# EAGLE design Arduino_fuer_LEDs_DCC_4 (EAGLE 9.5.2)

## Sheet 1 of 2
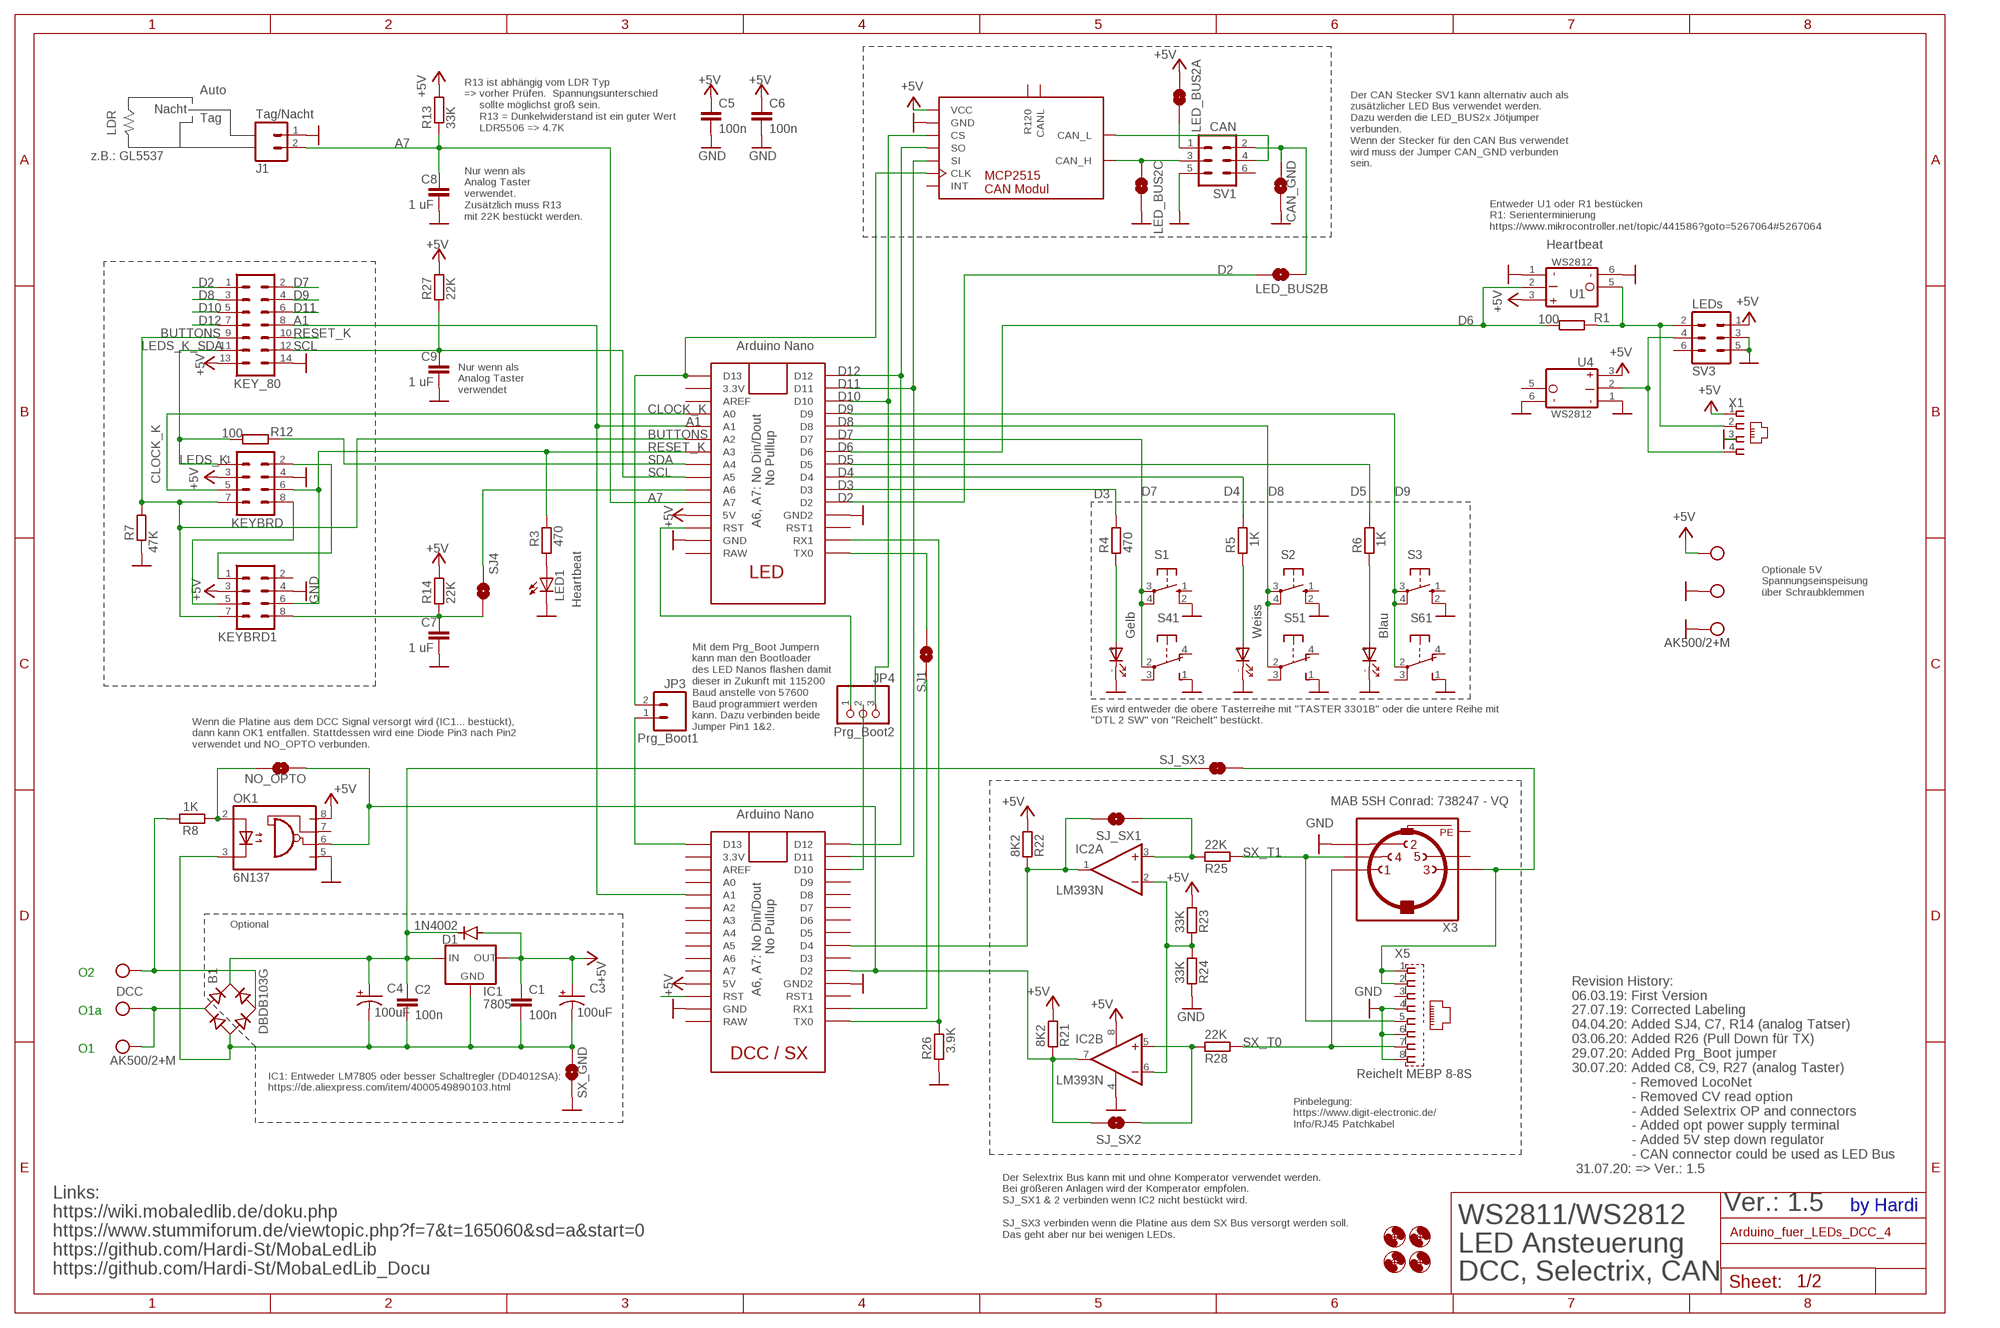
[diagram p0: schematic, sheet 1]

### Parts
B1  DBDB103G  DBDB10G  [DB]
C1  100n  C-EU025-025X050  [C025-025X050]
C2  100n  C-EU025-025X050  [C025-025X050]
C3  100uF  SPARKFUN-CAPACITORS_100UF-25V-20%(PTH)  [SPARKFUN-CAPACITORS_CPOL-RADIAL-100UF-25V]
C4  100uF  SPARKFUN-CAPACITORS_100UF-25V-20%(PTH)  [SPARKFUN-CAPACITORS_CPOL-RADIAL-100UF-25V]
C5  100n  C-EU025-025X050  [C025-025X050]
C6  100n  C-EU025-025X050  [C025-025X050]
C7  1 uF  C-EU025-025X050  [C025-025X050]
C8  1 uF  C-EU025-025X050  [C025-025X050]
C9  1 uF  C-EU025-025X050  [C025-025X050]
CAN2  MCP2515_CAN_MODUL  [MCP2515_CAN_MODUL]
CAN_GND  SOLDERJUMPERNO  [SJ_2S-NO]
D1  1N4002  1N4004  [DO41-10]
H1  MOUNT-HOLE3.0  [3,0]
H2  MOUNT-HOLE3.0  [3,0]
H3  MOUNT-HOLE3.0  [3,0]
H4  MOUNT-HOLE3.0  [3,0]
IC1  7805  78XXS  [78XXS]
IC2  LM393N  [DIL08]
J1  Tag/Nacht  M02PTH  [1X02]
JP3  Prg_Boot1  M02PTH  [1X02]
JP4  Prg_Boot2  PINHD-1X3CB  [1X03-CLEANBIG]
KEY_80  ML14  [ML14]
KEYBRD  CON-HARTING-ML_ML08  [CON-HARTING-ML_ML08]
KEYBRD1  CON-HARTING-ML_ML08  [CON-HARTING-ML_ML08]
LED1  Heartbeat  LED3MM  [LED3MM]
LED_BUS2A  SOLDERJUMPERNO  [SJ_2S-NO]
LED_BUS2B  SOLDERJUMPERNO  [SJ_2S-NO]
LED_BUS2C  SOLDERJUMPERNO  [SJ_2S-NO]
NO_OPTO  SOLDERJUMPERNO  [SJ_2S-NO]
OK1  6N137  [DIL08]
R1  100  R0204/7  [0204/7]
R3  470  R0204/7  [0204/7]
R4  470  R0204/7  [0204/7]
R5  1K  R0204/7  [0204/7]
R6  1K  R0204/7  [0204/7]
R7  47K  R0204/7  [0204/7]
R8  1K  R0204/7  [0204/7]
R12  100  R0204/7  [0204/7]
R13  33K  R0204/7  [0204/7]
R14  22K  R0204/7  [0204/7]
R21  8K2  R-EU_0207/2V  [0207/2V]
R22  8K2  R-EU_0207/2V  [0207/2V]
R23  33K  R-EU_0207/2V  [0207/2V]
R24  33K  R-EU_0207/2V  [0207/2V]
R25  22K  R-EU_0207/2V  [0207/2V]
R26  3.9K  R0204/7  [0204/7]
R27  22K  R0204/7  [0204/7]
R28  22K  R-EU_0207/2V  [0207/2V]
S1  10-XX  [B3F-10XX]
S2  10-XX  [B3F-10XX]
S3  10-XX  [B3F-10XX]
S4  Gelb  SRKL  [SRKL]
S5  Weiss  SRKL  [SRKL]
S6  Blau  SRKL  [SRKL]
SJ1  SOLDERJUMPERNO  [SJ_2S-NO]
SJ4  SOLDERJUMPERNO  [SJ_2S-NO]
SJ_SX1  SOLDERJUMPERNO  [SJ_2S-NO]
SJ_SX2  SOLDERJUMPERNO  [SJ_2S-NO]
SJ_SX3  SOLDERJUMPERNO  [SJ_2S-NO]
SV1  CAN  ML6  [ML6]
SV3  LEDs  ML6  [ML6]
SX_GND  SOLDERJUMPERNO  [SJ_2S-NO]
U1  WS2812_MODUL  [WS2812_LED_MODUL]
U2  LED NANO  NANO  [NANO]
U3  DCC NANO  NANO  [NANO]
U4  WS2812_MODUL  [WS2812_LED_MODUL]
X1  RJ10  [RJ10]
X2  AK500/2+M  [AK500/2+M]
X3  MAB 5SH Conrad: 738247 - VQ  MAB5SH  [MAB5SH]
X4  AK500/2+M  [AK500/2+M]
X5  Reichelt MEBP 8-8S  RJ45_MEBP8-8S  [RJ45_MEBP8-8S]

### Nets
+5V: C1.1 C3.1(+) C5.1 C6.1 CAN2.1(VCC) D1.A IC1.OUT IC2.8(P:V+) KEY_80.13 KEYBRD1.3 KEYBRD.3 LED_BUS2A.1 OK1.8(VCC) R13.2 R14.2 R21.2 R22.2 R23.2 R27.2 SV3.1 U1.3(VDD) U2.5V U3.5V U4.3(VDD) X1.1 X4.2
A1: KEY_80.8 U2.A1 U3.A1
A7: C8.1 J1.2 R13.1 U2.A7
BUTTONS: KEY_80.9 KEYBRD1.7 KEYBRD.7 R7.2 U2.A2
CAN_H: CAN2.9(CAN_H) LED_BUS2C.1 SV1.3
CAN_L: CAN2.8(CAN_L) SV1.4
CLOCK_K: KEYBRD.5 U2.A0
D2: KEY_80.1 LED_BUS2B.1 U2.D2
D3: R4.2 U2.D3
D4: R5.2 U2.D4
D5: R6.2 U2.D5
D6: R1.2 U1.2(DIN) U2.D6
D7: KEY_80.2 S1.3(P) S1.4(P1) S4.2(1:P) U2.D7
D8: KEY_80.3 S2.3(P) S2.4(P1) S5.2(1:P) U2.D8
D9: KEY_80.4 S3.3(P) S3.4(P1) S6.2(1:P) U2.D9
D10: CAN2.3(CS) JP4.3 KEY_80.5 U2.D10
D11: CAN2.5(SI) KEY_80.6 U2.D11 U3.D11
D12: CAN2.4(SO) KEY_80.7 U2.D12 U3.D12
GND: C5.2 C6.2 C7.2 C8.2 C9.2 CAN2.2(GND) CAN_GND.2 IC2.4(P:V-) J1.1 KEY_80.14 KEYBRD1.4 KEYBRD.4 LED1.K(C) LED_BUS2C.2 OK1.5(GND) R7.1 R24.1 R26.1 S1.2(S1) S2.2(S1) S3.2(S1) S4.1(1:S) S4.-(D1:C) S5.1(1:S) S5.-(D1:C) S6.1(1:S) S6.-(D1:C) SV1.5 SV3.3 SV3.5 SX_GND.2 U1.1(GND) U1.6(GND1) U2.GND U2.GND1(GND2) U3.GND U3.GND1(GND2) U4.1(GND) U4.6(GND1) X1.3 X3.2 X4.1 X4.M X5.4 X5.6 X5.8
LEDS_K_SDA: KEY_80.11 KEYBRD.1 R12.2
N$1: SJ1.2 U2.TX0
N$2: R1.1 SV3.2 U1.5(DO) X1.2
N$3: R26.2 U2.RX1 U3.TX0
N$4: R4.1 S4.+(D1:A)
N$5: CAN2.6(CLK) JP3.2 U2.D13
N$6: R5.1 S5.+(D1:A)
N$7: R6.1 S6.+(D1:A)
N$8: IC2.7(B:OUT) NO_OPTO.1 OK1.6(VO) R21.1 SJ_SX2.2 U3.D2
N$9: U3.RST
N$10: LED_BUS2A.2 SV1.1
N$11: SV3.4 U4.2(DIN) X1.4
N$12: B1.AC2 R8.2 X2.2
N$13: B1.AC1 X2.1 X2.M
N$14: B1.+ C2.1 C4.1(+) D1.C IC1.IN SJ_SX3.2
N$15: JP4.1 U2.RST
N$16: IC2.1(A:OUT) R22.1 SJ_SX1.2 U3.D4
N$17: B1.- C1.2 C2.2 C3.2(-) C4.2(-) IC1.GND OK1.3(C) SX_GND.1
N$18: SJ1.1 U3.RX1
N$19: LED1.A R3.1
N$20: JP3.1 U3.D13
N$21: NO_OPTO.2 OK1.2(A) R8.1
N$23: C7.1 KEYBRD1.8 R14.1 SJ4.2
N$24: KEYBRD1.1 KEYBRD.2
N$25: KEYBRD1.5 KEYBRD.8
N$26: SJ_SX3.1 X3.3 X5.1 X5.2
N$27: SJ4.1 U2.A6
N$28: JP4.2 U3.D10
N$29: CAN_GND.1 LED_BUS2B.2 SV1.2
N$38: IC2.2(A:-IN) IC2.6(B:-IN) R23.1 R24.2
N$39: IC2.3(A:+IN) R25.1 SJ_SX1.1
N$42: IC2.5(B:+IN) R28.1 SJ_SX2.1
RESET_K: KEY_80.10 KEYBRD1.6 KEYBRD.6 R3.2 U2.A3
SCL: C9.1 KEY_80.12 R27.1 U2.A5
SDA: R12.1 U2.A4
SX_T0: R28.2 X3.1 X5.7
SX_T1: R25.2 X3.4 X5.5
Unconnected: CAN2.7(INT) CAN2.10(R120) CAN2.11(CANL) KEYBRD1.2 OK1.7(VE) S1.1(S) S2.1(S) S3.1(S) S4.3(1:P) S4.4(1:O) S5.3(1:P) S5.4(1:O) S6.3(1:P) S6.4(1:O) SV1.6 SV3.6 U2.3.3V U2.AREF U2.RAW U2.RST1 U3.3.3V U3.A0 U3.A2 U3.A3 U3.A4 U3.A5 U3.A6 U3.A7 U3.AREF U3.D3 U3.D5 U3.D6 U3.D7 U3.D8 U3.D9 U3.RAW U3.RST1 U4.5(DO) X3.5 X5.3

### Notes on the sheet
- R13 ist abhängig vom LDR Typ
  => vorher Prüfen.  Spannungsunterschied
       sollte möglichst groß sein.
       R13 = Dunkelwiderstand ist ein guter Wert
       LDR5506 => 4.7K
- Der CAN Stecker SV1 kann alternativ auch als
  zusätzlicher LED Bus verwendet werden.
  Dazu werden die LED_BUS2x Jötjumper
  verbunden.
  Wenn der Stecker für den CAN Bus verwendet
  wird muss der Jumper CAN_GND verbunden
  sein.
- Auto
- Nacht
- Tag
- LDR
- z.B.: GL5537
- Nur wenn als
  Analog Taster
  verwendet.
  Zusätzlich muss R13 
  mit 22K bestückt werden.
- Entweder U1 oder R1 bestücken 
  R1: Serienterminierung
  https://www.mikrocontroller.net/topic/441586?goto=5267064#5267064
- Heartbeat
- Nur wenn als
  Analog Taster
  verwendet
- LEDS_K
- A6, A7: No Din/Dout 
              No Pullup
- LED
- Optionale 5V
  Spannungseinspeisung
  über Schraubklemmen
- Es wird entweder die obere Tasterreihe mit "TASTER 3301B" oder die untere Reihe mit 
  "DTL 2 SW" von "Reichelt" bestückt.
- Wenn die Platine aus dem DCC Signal versorgt wird (IC1... bestückt), 
  dann kann OK1 entfallen. Stattdessen wird eine Diode Pin3 nach Pin2
  verwendet und NO_OPTO verbunden.
- Mit dem Prg_Boot Jumpern
  kann man den Bootloader
  des LED Nanos flashen damit
  dieser in Zukunft mit 115200
  Baud anstelle von 57600
  Baud programmiert werden 
  kann. Dazu verbinden beide
  Jumper Pin1 1&2.
- Optional
- O2
- DCC
- A6, A7: No Din/Dout 
              No Pullup
- O1a
- DCC / SX
- O1
- IC1: Entweder LM7805 oder besser Schaltregler (DD4012SA):
  https://de.aliexpress.com/item/4000549890103.html
- Pinbelegung:
  https://www.digit-electronic.de/
  Info/RJ45 Patchkabel
- Der Selextrix Bus kann mit und ohne Komperator verwendet werden.
  Bei größeren Anlagen wird der Komperator empfolen. 
  SJ_SX1 & 2 verbinden wenn IC2 nicht bestückt wird.
  
  SJ_SX3 verbinden wenn die Platine aus dem SX Bus versorgt werden soll.
  Das geht aber nur bei wenigen LEDs.
- Revision History:
  06.03.19: First Version
  27.07.19: Corrected Labeling
  04.04.20: Added SJ4, C7, R14 (analog Tatser)
  03.06.20: Added R26 (Pull Down für TX)
  29.07.20: Added Prg_Boot jumper
  30.07.20: Added C8, C9, R27 (analog Taster)
                 - Removed LocoNet
                 - Removed CV read option
                 - Added Selextrix OP and connectors
                 - Added opt power supply terminal 
                 - Added 5V step down regulator
                 - CAN connector could be used as LED Bus
   31.07.20: => Ver.: 1.5
- Ver.: 1.5 | by Hardi
- Links:
  https://wiki.mobaledlib.de/doku.php
  https://www.stummiforum.de/viewtopic.php?f=7&t=165060&sd=a&start=0
  https://github.com/Hardi-St/MobaLedLib
  https://github.com/Hardi-St/MobaLedLib_Docu
- WS2811/WS2812
  LED Ansteuerung
  DCC, Selectrix, CAN

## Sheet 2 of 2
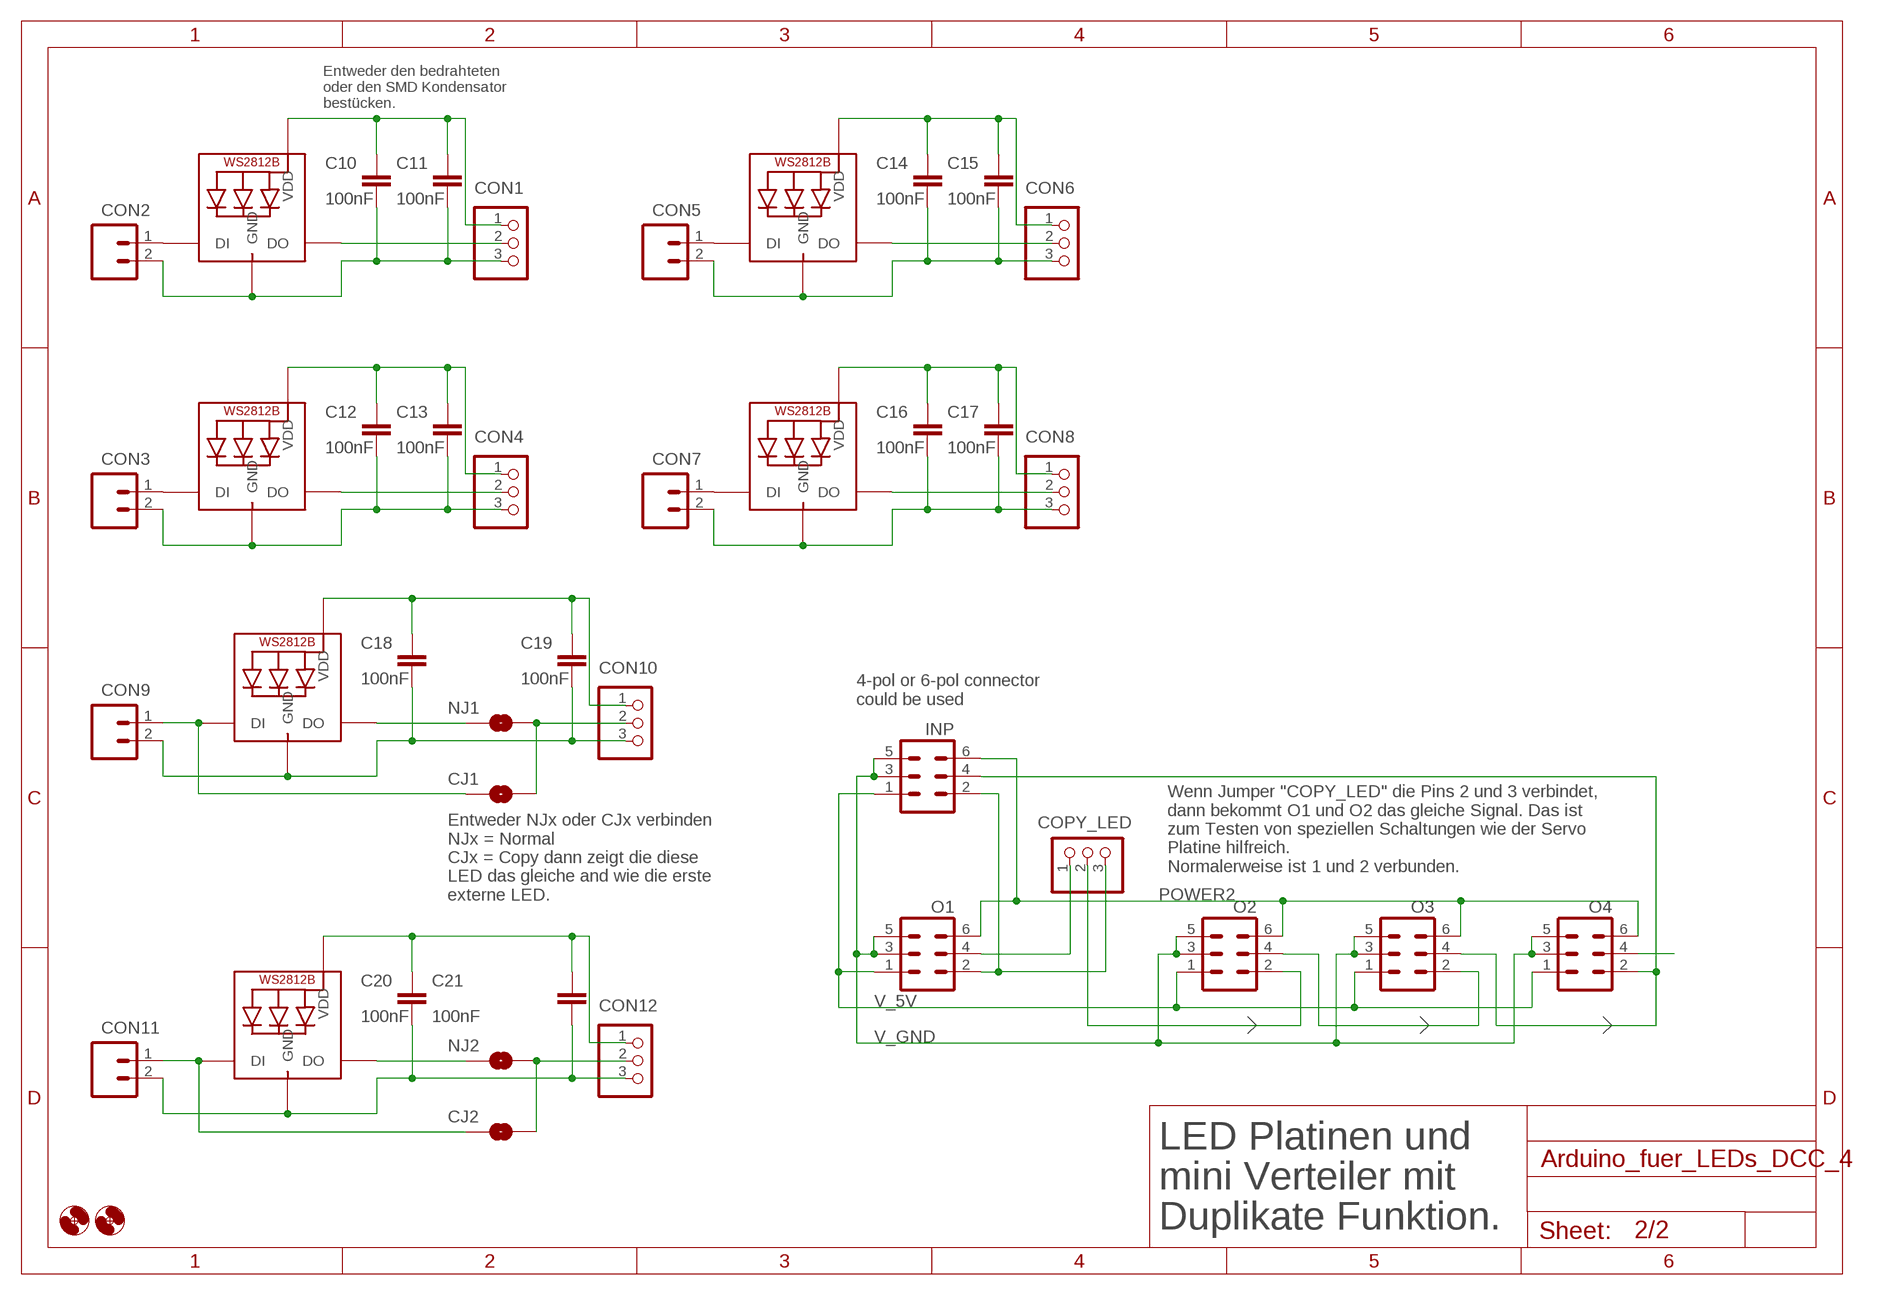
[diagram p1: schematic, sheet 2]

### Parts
C10  100nF  C-EU025-025X050  [C025-025X050]
C11  100nF  C-EUC1206  [C1206]
C12  100nF  C-EU025-025X050  [C025-025X050]
C13  100nF  C-EUC1206  [C1206]
C14  100nF  C-EU025-025X050  [C025-025X050]
C15  100nF  C-EUC1206  [C1206]
C16  100nF  C-EU025-025X050  [C025-025X050]
C17  100nF  C-EUC1206  [C1206]
C18  100nF  C-EU025-025X050  [C025-025X050]
C19  100nF  C-EUC1206  [C1206]
C20  100nF  C-EU025-025X050  [C025-025X050]
C21  100nF  C-EUC1206  [C1206]
CJ1  SOLDERJUMPERNO  [SJ_2S-NO]
CJ2  SOLDERJUMPERNO  [SJ_2S-NO]
CON1  PINHD-1X3CB  [1X03-CLEANBIG]
CON2  M02PTH  [1X02]
CON3  M02PTH  [1X02]
CON4  PINHD-1X3CB  [1X03-CLEANBIG]
CON5  M02PTH  [1X02]
CON6  PINHD-1X3CB  [1X03-CLEANBIG]
CON7  M02PTH  [1X02]
CON8  PINHD-1X3CB  [1X03-CLEANBIG]
CON9  M02PTH  [1X02]
CON10  PINHD-1X3CB  [1X03-CLEANBIG]
CON11  M02PTH  [1X02]
CON12  PINHD-1X3CB  [1X03-CLEANBIG]
COPY_LED  PINHD-1X3CB  [1X03-CLEANBIG]
H5  MOUNT-HOLE3.0  [3,0]
H6  MOUNT-HOLE3.0  [3,0]
INP  ML6  [ML6]
LED2  WS2812B5050  [WS2812B]
LED3  WS2812B5050  [WS2812B]
LED4  WS2812B3535  [LED3535]
LED5  WS2812B3535  [LED3535]
LED6  WS2812B5050  [WS2812B]
LED7  WS2812B3535  [LED3535]
NJ1  SOLDERJUMPERNO  [SJ_2S-NO]
NJ2  SOLDERJUMPERNO  [SJ_2S-NO]
O1  ML6  [ML6]
O2  ML6  [ML6]
O3  ML6  [ML6]
O4  ML6  [ML6]

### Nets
N$22: C10.2 C11.2 CON1.3 CON2.2 LED2.3-GND(GND)
N$30: CON1.2 LED2.2-DOUT(DO)
N$31: C12.2 C13.2 CON3.2 CON4.3 LED3.3-GND(GND)
N$32: C10.1 C11.1 CON1.1 LED2.1-VDD(VDD)
N$33: CON2.1 LED2.4-DIN(DI)
N$34: CON4.2 LED3.2-DOUT(DO)
N$35: C12.1 C13.1 CON4.1 LED3.1-VDD(VDD)
N$36: CON3.1 LED3.4-DIN(DI)
N$37: C14.2 C15.2 CON5.2 CON6.3 LED4.4(GND)
N$40: CON6.2 LED4.3(DO)
N$41: C14.1 C15.1 CON6.1 LED4.2(VDD)
N$43: CON5.1 LED4.1(DI)
N$44: C16.2 C17.2 CON7.2 CON8.3 LED5.4(GND)
N$45: CON8.2 LED5.3(DO)
N$46: C16.1 C17.1 CON8.1 LED5.2(VDD)
N$47: CON7.1 LED5.1(DI)
N$48: C18.2 C19.2 CON9.2 CON10.3 LED6.3-GND(GND)
N$49: LED6.2-DOUT(DO) NJ1.1
N$50: C18.1 C19.1 CON10.1 LED6.1-VDD(VDD)
N$51: CJ1.1 CON9.1 LED6.4-DIN(DI)
N$52: INP.4 O3.4 O4.2
N$53: O4.4
N$54: C20.2 C21.2 CON11.2 CON12.3 LED7.4(GND)
N$55: COPY_LED.2 O2.2
N$56: LED7.3(DO) NJ2.1
N$57: COPY_LED.3 INP.2 O1.2
N$58: O2.4 O3.2
N$59: C20.1 C21.1 CON12.1 LED7.2(VDD)
N$60: COPY_LED.1 O1.4
N$61: CJ2.1 CON11.1 LED7.1(DI)
N$62: CJ2.2 CON12.2 NJ2.2
N$63: CJ1.2 CON10.2 NJ1.2
POWER2: INP.6 O1.6 O2.6 O3.6 O4.6
V_5V: INP.1 O1.1 O2.1 O3.1 O4.1
V_GND: INP.3 INP.5 O1.3 O1.5 O2.3 O2.5 O3.3 O3.5 O4.3 O4.5

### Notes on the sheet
- Entweder den bedrahteten 
  oder den SMD Kondensator 
  bestücken.
- 4-pol or 6-pol connector
  could be used
- Wenn Jumper "COPY_LED" die Pins 2 und 3 verbindet,
  dann bekommt O1 und O2 das gleiche Signal. Das ist
  zum Testen von speziellen Schaltungen wie der Servo 
  Platine hilfreich.
  Normalerweise ist 1 und 2 verbunden.
- Entweder NJx oder CJx verbinden
  NJx = Normal
  CJx = Copy dann zeigt die diese
  LED das gleiche and wie die erste
  externe LED.
- LED Platinen und
  mini Verteiler mit 
  Duplikate Funktion.

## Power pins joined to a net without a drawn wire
PE: X3.PE X3.PE@(PE)

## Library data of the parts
B1 = Arduino_fuer_LEDs_DCC_2:DB?*G: Single Phase 1.0 AMP Glass Passivated Bridge Rectifier Taiwan Semiconductor Co.,Ltd. - TSC Source: http://www.taiwansemi.com/TSCbig5/ezcatfiles/cust/img/img/db101g.pdf http://www.ts.com.tw/db/pictures/modules/PDT/PDT060207001/DBLS201G.pdf
C1 C2 C5-C21 = rcl:C-EU: CAPACITOR, European symbol
C3 C4 = Sound_MP3-TF-16P_and_WS2811:SPARKFUN-CAPACITORS_100UF-25V-20%(PTH): CAP-08439; PROD_ID: CAP-08439
CAN2 = Arduino_fuer_LEDs_DCC_2_All:MCP2515_CAN_MODUL: MCP2515 CAN Modul
CAN_GND CJ1 CJ2 LED_BUS2A LED_BUS2B LED_BUS2C NJ1 NJ2 NO_OPTO SJ1 SJ4 SJ_SX1-SJ_SX3 SX_GND = SparkFun-Retired:SOLDERJUMPER: Solder Jumper
CON1 CON4 CON6 CON8 CON10 CON12 COPY_LED JP4 = adafruit:PINHD-1X3: PIN HEADER
CON2 CON3 CON5 CON7 CON9 CON11 J1 JP3 = SparkFun-Connectors:M02: Standard 2-pin 0.1" header. Use with
D1 = diode:1N4004: DIODE
H1-H6 = holes:MOUNT-HOLE: MOUNTING HOLE with drill center marker
IC1 = v-reg:78XXS: VOLTAGE REGULATOR
IC2 = linear:LM393: COMPARATOR
INP O1-O4 = con-harting-ml:ML6: HARTING; OC_FARNELL: unknown; OC_NEWARK: unknown
KEY_80 = Arduino_fuer_LEDs_DCC_2:ML14: HARTING; OC_FARNELL: unknown; OC_NEWARK: unknown
KEYBRD KEYBRD1 = PushButtonAction_4017_2:CON-HARTING-ML_ML08: Modified by Hardi; OC_FARNELL: unknown; OC_NEWARK: unknown
LED1 = Arduino_fuer_LEDs_DCC_2:LED: LED
LED2-LED7 = adafruit:WS2812B
OK1 = Arduino_fuer_LEDs_DCC_2:6N137: MOTOROLA OPTO COUPLER; MPN: 6N137; OC_FARNELL: 1328376; OC_NEWARK: 52M1895
R1 R3-R8 R12-R14 R26 R27 = Arduino_fuer_LEDs_DCC_2:R: RESISTOR, European symbol; SPICEMODEL: NONE; SPICEPREFIX: R
R21-R25 R28 = rcl:R-EU_: RESISTOR, European symbol
S1-S3 = switch-omron:10-XX: OMRON SWITCH; MPN: B3F-1000; OC_FARNELL: 176432; OC_NEWARK: 36M3542
S4-S6 = switch-misc:SRKL: SWITCH
SV1 SV3 = Arduino_fuer_LEDs_DCC_2:ML6: HARTING; OC_FARNELL: unknown; OC_NEWARK: unknown
U1 U4 = Arduino_fuer_LEDs_DCC_2_All:WS2812_MODUL: WS2812 Modul mit Winkelsteckern (by Hardi)
U2 U3 = Arduino_fuer_LEDs_DCC_2:NANO: Arduino Nano
X1 = RJ10:RJ10: RJ10 Connector "C:\Dat\Märklin\Schaltpläne\Allgemein\RJ10_Stecker_Layout.docx" ...; OC_FARNELL: unknown; OC_NEWARK: unknown
X2 X4 = Arduino_fuer_LEDs_DCC_2:AK500/2+M
X3 = con-hirschmann:MAB5SH: Female CONNECTOR 5 pins 90 deg. with shield, horizontal (DIN 41524); OC_FARNELL: 809883; OC_NEWARK: unknown
X5 = RJ45_Reichelt:RJ45_MEBP8-8S: AMP connector

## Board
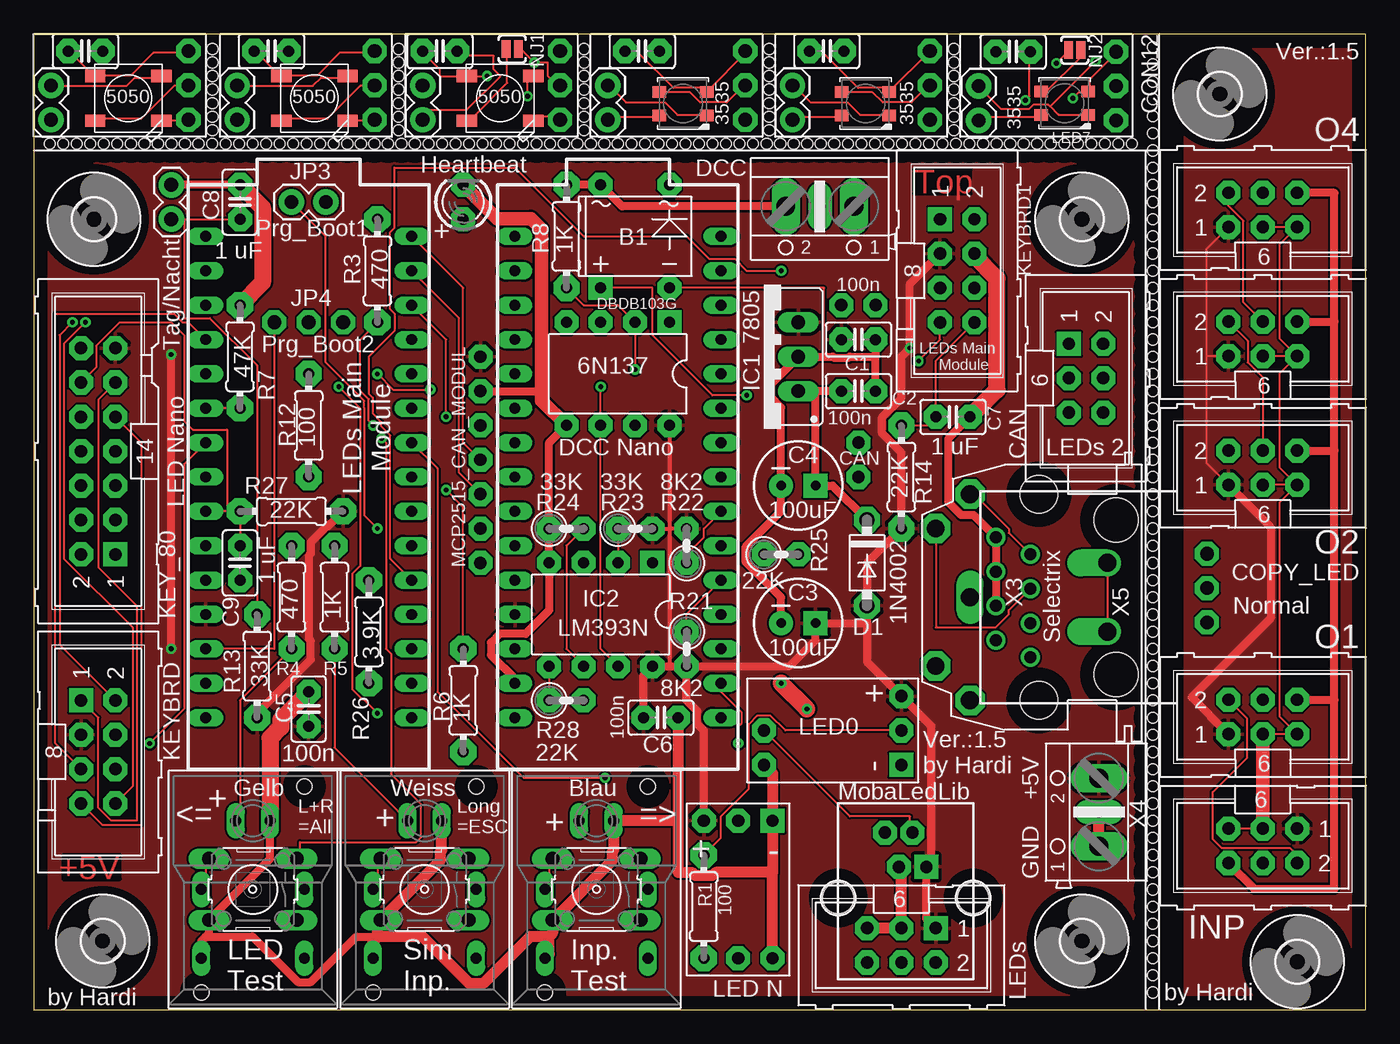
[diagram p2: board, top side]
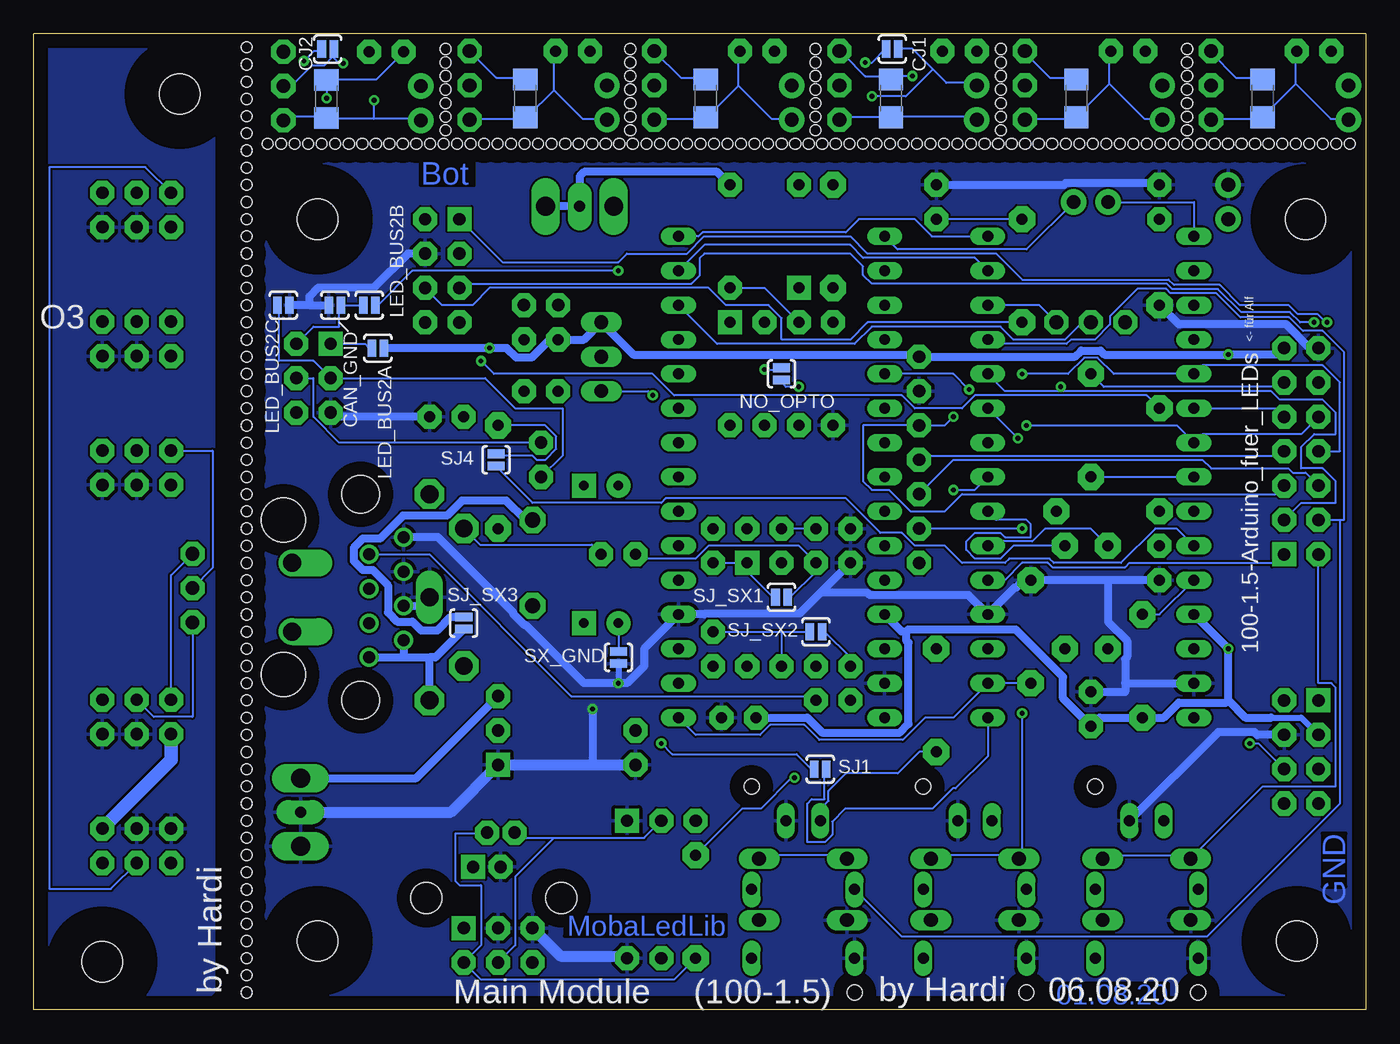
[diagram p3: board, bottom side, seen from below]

Size 98.46 x 72.12 mm. Coordinates in mm from the lower left corner, seen from the top.
Outline: 13.76,72.12 26.46,72.12
Outline: 27.48,72.12 40.18,72.12
Outline: 0,72.12 0,0 98.46,0 98.46,72.12 0,72.12
Copper layers (1*16): Top 0.035mm / dielectric 1.5mm / Bottom 0.035mm
Design rules "default": minimum track width 6mil, minimum drill 0.35mm, track to track 6mil, track to pad 6mil, pad to pad 6mil, via to via 6mil, smd to smd 6mil, copper to edge 40mil, drill to drill 6mil, minimum pad ring 10mil, minimum via ring 8mil, stop-mask expansion 4mil, vias tented up to drill 0mil, thermal gap 10mil
Holes 0.8 mm at 82.72,1.27 82.72,2.54 82.72,3.81 82.72,5.08 82.72,6.35 82.72,7.62 82.72,8.89 82.72,10.16 82.72,11.43 82.72,12.7 82.72,13.97 82.72,15.24 82.72,16.51 82.72,17.78 82.72,19.05 82.72,20.32 82.72,21.59 82.72,22.86 82.72,24.13 82.72,25.4 82.72,26.67 82.72,27.94 82.72,29.21 82.72,30.48 82.72,31.75 82.72,33.02 82.72,34.29 82.72,35.56 82.72,36.83 82.72,38.1 82.72,39.37 82.72,40.64 82.72,41.91 82.72,43.18 82.72,44.45 82.72,45.72 82.72,46.99 82.72,48.26 82.72,49.53 82.72,50.8 82.72,52.07 82.72,53.34 82.72,54.61 82.72,55.88 82.72,57.15 82.72,58.42 82.72,59.69 82.72,60.96 82.72,62.23 82.72,63.5 82.72,64.77 82.72,66.04 82.72,67.31 82.72,68.58 82.72,69.85 82.72,71.12 1.18,64 2.17,64 3.17,64 4.17,64 5.17,64 6.17,64 7.17,64 8.18,64 9.18,64 10.18,64 11.18,64 12.18,64 13.18,64 14.18,64 15.18,64 16.18,64 17.18,64 18.18,64 19.18,64 20.18,64 21.18,64 22.18,64 23.18,64 24.18,64 25.18,64 26.18,64 27.18,64 28.18,64 29.18,64 30.18,64 31.18,64 32.17,64 33.17,64 34.17,64 35.17,64 36.17,64 37.17,64 38.17,64 39.17,64 40.17,64 41.17,64 42.17,64 43.17,64 44.17,64 45.17,64 46.17,64 47.17,64 48.17,64 49.17,64 50.17,64 51.17,64 52.17,64 53.17,64 54.17,64 55.17,64 56.17,64 57.17,64 58.17,64 59.17,64 60.17,64 61.17,64 62.17,64 63.17,64 64.17,64 65.17,64 66.17,64 67.17,64 68.17,64 69.17,64 70.17,64 71.17,64 72.17,64 73.17,64 74.17,64 75.17,64 76.17,64 77.17,64 78.17,64 79.17,64 80.17,64 81.17,64 13.2,65 13.2,66 13.2,67 13.2,68 13.2,69 13.2,70 13.2,71 26.96,65 26.96,66 26.96,67 26.96,68 26.96,69 26.96,70 26.96,71 40.68,65 40.68,66 40.68,67 40.68,68 40.68,69 40.68,70 40.68,71 54.36,65 54.36,66 54.36,67 54.36,68 54.36,69 54.36,70 54.36,71 68.02,65 68.02,66 68.02,67 68.02,68 68.02,69 68.02,70 68.02,71

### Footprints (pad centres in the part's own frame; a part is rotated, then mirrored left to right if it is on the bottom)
DB = drill 0.813 pad 1.778 square: + -2.54,-3.81 | drill 0.813 pad 1.778 octagon: - 2.54,-3.81; AC1 2.54,3.81; AC2 -2.54,3.81
C025-025X050 = drill 0.813 pad 1.778 octagon: 1 -1.27,0; 2 1.27,0
SPARKFUN-CAPACITORS_CPOL-RADIAL-100UF-25V = drill 0.7 pad 1.778 square: 1 1.27,0 | drill 0.7 pad 1.778: 2 -1.27,0
C1206 = smd 1.6 x 1.8: 1 -1.4,0; 2 1.4,0
MCP2515_CAN_MODUL = drill 0.914 pad 1.778 octagon: 1 0,0; 2 0,-2.54; 3 0,-5.08; 4 0,-7.62; 5 0,-10.16; 6 0,-12.7; 7 0,-15.24; 8 27.94,-6.35; 9 27.94,-8.89; 10 26.67,3.81; 11 29.21,3.81
SJ_2S-NO = smd 0.635 x 1.27: 1 -0.45,0; 2 0.45,0
1X03-CLEANBIG = drill 1.016 pad 1.778 octagon: 1 -2.54,0; 2 0,0; 3 2.54,0
1X02 = drill 1.016 pad 1.88: 1 0,0; 2 2.54,0
DO41-10 = drill 1.118 pad 1.93 octagon: A 3.175,0; C -3.175,0
3,0 = hole 3: 0,0
78XXS = drill 1.016 long: GND 0,-2.54; IN -2.54,-2.54; OUT 2.54,-2.54
DIL08 = drill 0.813 pad 1.778 square: 1 -3.81,-3.81 | drill 0.813 pad 1.778 octagon: 2 -1.27,-3.81; 3 1.27,-3.81; 4 3.81,-3.81; 5 3.81,3.81; 6 1.27,3.81; 7 -1.27,3.81; 8 -3.81,3.81
ML6 = drill 0.914 pad 1.778 octagon: 1 -2.54,-1.27; 2 -2.54,1.27; 3 0,-1.27; 4 0,1.27; 5 2.54,-1.27; 6 2.54,1.27
ML14 = drill 0.914 pad 1.778 square: 1 -7.62,-1.27 | drill 0.914 pad 1.778 octagon: 2 -7.62,1.27; 3 -5.08,-1.27; 4 -5.08,1.27; 5 -2.54,-1.27; 6 -2.54,1.27; 7 0,-1.27; 8 0,1.27; 9 2.54,-1.27; 10 2.54,1.27; 11 5.08,-1.27; 12 5.08,1.27; 13 7.62,-1.27; 14 7.62,1.27
CON-HARTING-ML_ML08 = drill 0.914 pad 1.778 square: 1 -5.08,-1.27 | drill 0.914 pad 1.778 octagon: 2 -5.08,1.27; 3 -2.54,-1.27; 4 -2.54,1.27; 5 0,-1.27; 6 0,1.27; 7 2.54,-1.27; 8 2.54,1.27
LED3MM = drill 0.813 pad 1.778 octagon: A -1.27,0; K 1.27,0
WS2812B = smd 1.5 x 0.9: 1-VDD 2.45,-1.65; 2-DOUT 2.45,1.65; 3-GND -2.45,1.65; 4-DIN -2.45,-1.65
LED3535 = smd 1 x 0.85: 1 -1.75,0.875; 2 -1.75,-0.875; 3 1.75,-0.875; 4 1.75,0.875
0204/7 = drill 0.813 pad 1.93 octagon: 1 -3.81,0; 2 3.81,0
0207/2V = drill 0.813 pad 1.778 octagon: 1 -1.27,0; 2 1.27,0
B3F-10XX = drill 1.016 long: 1 -3.251,2.261; 2 3.251,2.261; 3 -3.251,-2.261; 4 3.251,-2.261
SRKL = drill 0.813 long: 1 -3.81,-5.08; 2 -3.81,0; 3 3.81,0; 4 3.81,-5.08; + -1.27,5.08; - 1.27,5.08 | hole 1.118: 3.81,7.62; -3.81,-7.62
ML6' = drill 0.914 pad 1.778 square: 1 -2.54,-1.27 | drill 0.914 pad 1.778 octagon: 2 -2.54,1.27; 3 0,-1.27; 4 0,1.27; 5 2.54,-1.27; 6 2.54,1.27
WS2812_LED_MODUL = drill 0.914 pad 1.778 square: 1 -5.08,-5.08 | drill 0.914 pad 1.778 octagon: 2 -2.54,-5.08; 3 0,-5.08; 5 -2.54,5.08; 6 -5.08,5.08
NANO = drill 0.8 long: 3.3V -10.16,24.13; 5V -10.16,-1.27; A0 -10.16,19.05; A1 -10.16,16.51; A2 -10.16,13.97; A3 -10.16,11.43; A4 -10.16,8.89; A5 -10.16,6.35; A6 -10.16,3.81; A7 -10.16,1.27; AREF -10.16,21.59; D2 5.08,1.27; D3 5.08,3.81; D4 5.08,6.35; D5 5.08,8.89; D6 5.08,11.43; D7 5.08,13.97; D8 5.08,16.51; D9 5.08,19.05; D10 5.08,21.59; D11 5.08,24.13; D12 5.08,26.67; D13 -10.16,26.67; GND -10.16,-6.35; GND1 5.08,-1.27; RAW -10.16,-8.89; RST -10.16,-3.81; RST1 5.08,-3.81; RX1 5.08,-6.35; TX0 5.08,-8.89
RJ10 = drill 0.9 pad 1.778 square: 1 -1.524,-2.3 | drill 0.9 pad 1.778 octagon: 2 -0.508,-4.84; 3 0.508,-2.3; 4 1.524,-4.84 | hole 2.3: 5,0; -5,0
AK500/2+M = drill 1.397 long: 1 -2.515,0; 2 2.515,0 | drill 0.813 pad 1.778 long: M 0,0
MAB5SH = drill 1.321 pad 2.184 octagon: 1 7.62,5.08; 3 -7.62,5.08; 4 5.08,7.62; 5 -5.08,7.62 | drill 1.321 long: 2 0,5.08 | drill 1.321 offset: PE -2.54,-5.08; PE@ 2.54,-5.08 | hole 2.794: 7.62,0; -7.62,0
RJ45_MEBP8-8S = drill 0.889: 1 -4.445,6.35; 2 -3.175,8.89; 3 -1.905,6.35; 4 -0.635,8.89; 5 0.635,6.35; 6 1.905,8.89; 7 3.175,6.35; 8 4.445,8.89 | hole 3.251: -5.715,0; 5.715,0

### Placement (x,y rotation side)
B1  44.45,57.15 0 top
C1  60.96,49.53 0 top
C2  60.96,45.72 0 top
C3  56.52,28.57 0 top
C4  56.52,38.73 0 top
C5  20.32,22.23 90 top
C6  46.35,21.59 0 top
C7  67.94,43.81 0 top
C8  15.24,59.69 90 top
C9  15.24,33.02 270 top
C10  3.81,70.85 0 top
C11  7.62,67.36 270 bottom
C12  17.57,70.85 0 top
C13  21.38,67.36 270 bottom
C14  44.97,70.85 0 top
C15  48.78,67.36 270 bottom
C16  58.63,70.85 0 top
C17  62.12,67.36 270 bottom
C18  30.02,70.85 0 top
C19  35.1,67.36 270 bottom
C20  72.39,70.8 0 top
C21  76.83,67.31 270 bottom
CAN2  33.02,48.26 0 top
CAN_GND  76.2,52.07 180 bottom
CJ1  35,71 180 bottom
CJ2  76.73,71 0 bottom
CON1  11.43,68.31 270 top
CON2  1.27,68.31 270 top
CON3  15.03,68.31 270 top
CON4  25.19,68.31 270 top
CON5  42.43,68.31 270 top
CON6  52.59,68.31 270 top
CON7  56.09,68.31 270 top
CON8  66.25,68.31 270 top
CON9  28.75,68.31 270 top
CON10  38.91,68.31 270 top
CON11  69.85,68.26 270 top
CON12  80.01,68.26 270 top
COPY_LED  86.72,31.16 90 top
D1  61.59,33.02 270 top
H1  5.08,5.08 0 top
H2  4.45,58.42 0 top
H3  77.47,58.42 0 top
H4  77.47,5.08 0 top
H5  93.39,3.54 0 top
H6  87.68,67.67 0 top
IC1  53.98,48.26 90 top
IC2  41.91,29.21 180 top
INP  90.85,12.11 180 top
J1  10.16,60.96 270 top
JP3  21.59,59.69 180 top
JP4  20.32,50.8 0 top
KEY_80  4.76,41.27 90 top
KEYBRD  4.76,17.78 270 top
KEYBRD1  68.26,53.34 270 top
LED1  31.75,59.69 90 top
LED2  6.99,67.36 180 top
LED3  20.75,67.36 180 top
LED4  47.99,66.96 180 top
LED5  61.48,66.96 180 top
LED6  34.47,67.36 180 top
LED7  76.2,66.99 180 top
LED_BUS2A  73.03,48.9 180 bottom
LED_BUS2B  73.66,52.07 180 bottom
LED_BUS2C  80.01,52.07 0 bottom
NJ1  35.37,71 0 top
NJ2  76.95,70.92 180 top
NO_OPTO  43.18,46.99 90 bottom
O1  90.85,21.64 0 top
O2  90.85,40.05 0 top
O3  90.85,49.58 0 top
O4  90.85,59.1 0 top
OK1  43.18,46.99 180 top
R1  49.53,7.62 90 top
R3  25.4,54.61 270 top
R4  19.05,30.48 90 top
R5  22.23,30.48 90 top
R6  31.75,22.86 90 top
R7  15.24,48.26 270 top
R8  39.37,57.15 90 top
R12  20.32,43.18 90 top
R13  16.51,25.4 270 top
R14  64.14,39.37 270 top
R21  48.26,26.67 270 top
R22  48.26,34.29 90 top
R23  44.45,35.56 0 top
R24  39.37,35.56 0 top
R25  55.24,33.66 0 top
R26  24.77,27.94 270 top
R27  19.05,36.83 0 top
R28  39.37,22.86 0 top
S1  16.19,8.89 180 top
S2  28.89,8.89 180 top
S3  41.59,8.89 180 top
S4  16.19,8.89 0 top
S5  28.89,8.89 0 top
S6  41.59,8.89 0 top
SJ1  40.32,17.78 0 bottom
SJ4  64.29,40.64 90 bottom
SJ_SX1  43.18,30.48 180 bottom
SJ_SX2  40.64,27.94 180 bottom
SJ_SX3  66.67,28.57 90 bottom
SV1  CAN  [ML6']  77.79,46.67 270 top
SV3  LEDs  [ML6']  64.14,4.76 180 top
SX_GND  55.24,26.04 270 bottom
U1  59.05,23.18 90 top
U2  22.86,30.48 0 top
U3  45.72,30.48 0 top
U4  49.53,8.89 180 top
X1  64.45,8.26 180 top
X2  58.1,59.37 180 top
X3  74.3,30.48 90 top
X4  78.74,14.61 90 top
X5  80.01,30.48 90 top

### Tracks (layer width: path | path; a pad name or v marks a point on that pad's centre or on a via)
+5V  (via drill 0.35)
  Top 0.305: R23.2 46.99,35.56 | R22.2 46.99,35.56 | OK1.8 46.99,35.56 | 46.99,35.56 46.99,25.4
  Top 0.61: 61.59,28.57 C3.1 57.78,27.3 55.88,25.4 R21.2 | 61.59,28.57 D1.A 61.59,33.02 R14.2 64.14,41.17 62.71,42.59 62.71,43.77 64.14,45.19 64.14,48.26 v64.77,48.9 64.77,53.66 KEYBRD1.3 | 61.59,28.57 61.59,25.72 U1.3 66.36,20.95 66.36,11.11 65.98,10.73 X1.1 65.98,6.73 SV3.1 | R27.2 21.74,35.71 21.64,35.71 20.47,34.55 20.47,33.7 20.32,33.55 20.32,27.41 20.47,27.26 20.47,25.87 16.51,21.91 R13.2 | C6.1 45.09,24.77 IC2.8 46.99,25.4 R21.2 | U4.3 49.53,20.64 49.03,21.13 49.03,22.09 48.26,22.86 R21.2 | v10.16,26.67 v10.16,48.42
  Bottom 0.457: KEYBRD.3 4.76,21.59 6.99,21.59
  Bottom 0.61: LED_BUS2A.1 v64.77,48.9 63.5,48.9 62.79,48.18 61.67,48.18 60.33,49.53 C1.1 57.78,49.53 IC1.OUT 54.13,48.42 33.18,48.42 CAN2.1 21.49,48.26 21.04,48.72 19.61,48.72 19.31,48.42 v10.16,48.42 6.51,48.42 KEY_80.13 | U3.5V 34.29,27.94 33.97,27.94 | 33.97,27.94 33.82,28.09 25.87,28.09 22.38,24.61 22.38,23.02 C5.1 19.68,21.59 R13.2 14.93,21.59 13.81,22.7 10.32,22.7 10.16,22.86 | 33.97,27.94 33.97,27.31 33.8,27.13 33.8,21.13 34.45,20.48 40.16,20.48 41.27,21.59 C6.1 | X4.2 70.19,17.12 U1.3 | U2.5V v10.16,26.67 10.16,22.86 | 10.16,22.86 8.89,21.59 6.99,21.59
  pour Top: 0,60.96 2.54,63.5 3.81,63.5 82.55,63.5 82.55,5.08 81.28,3.81 77.47,0 0,0
A1  (via drill 0.35)
  Top 0.152: v25.4,46.99 26.56,45.83 v29.32,45.83
  Bottom 0.152: KEY_80.8 1.91,41.27 1.91,46.35 3.17,47.62 12.06,47.62 U2.A1 18.63,46.99 19.83,48.18 20.81,48.18 22.01,46.99 v25.4,46.99 | v29.32,45.83 30.48,46.99 U3.A1
A7
  Top 0.152: J1.2 11.11,58.42 | 11.11,58.42 C8.1 | R13.1 16.51,47.62 13.02,51.12 11.11,51.12 11.11,58.42
  Bottom 0.152: U2.A7 15.24,29.21 R13.1
BUTTONS  (via drill 0.35)
  Top 0.152: KEYBRD.7 5.08,13.65 7.94,13.65 7.94,41.91 KEY_80.9 | R7.2 U2.A2 | v65.41,47.94 66.99,49.53 KEYBRD1.7
  Bottom 0.152: v65.41,47.94 64.45,46.99 52.7,46.99 51.12,45.4 34.29,45.4 33.34,44.45 29.84,44.45 28.89,45.4 16.19,45.4 R7.2 | KEY_80.9 6.67,44.45 U2.A2
CAN_H
  Bottom 0.152: LED_BUS2C.1 80.33,52.07 80.33,47.94 77.79,47.94 SV1.3 65.09,46.67 62.87,44.45 59.37,44.45 59.37,40.96 CAN2.9
CAN_L
  Bottom 0.152: SV1.4 77.79,46.67 77.79,43.81 75.88,41.91 CAN2.8
CLOCK_K
  Top 0.152: KEYBRD.5 1.59,19.68 1.59,51.44 10.36,51.44 10.99,50.81 11.42,50.81 U2.A0
D2  (via drill 0.35)
  Top 0.152: U2.D2 26.35,33.34 26.35,42.45 25.69,43.11 25.69,43.43 25.06,44.06 25.06,45.24 24.77,45.53 24.77,48.26 26.67,50.16 26.67,51.44 26.35,51.75 26.35,57.47 26.67,57.78 26.67,62.23 35.56,62.23 40.64,57.15 48.26,57.15 49.92,55.49 51.82,55.49 52.7,54.61 v55.24,54.61
  Bottom 0.152: v55.24,54.61 70.48,54.61 73.03,52.07 LED_BUS2B.1 | KEY_80.1 6.67,33.02 17.46,33.02 17.78,32.7 23.18,32.7 23.5,33.02 25.4,33.02 26.67,31.75 U2.D2
D3
  Bottom 0.152: U2.D3 27.62,34.61 24.65,34.61 23.7,35.56 20.32,35.56 R4.2
D4
  Bottom 0.152: U2.D4 27.3,36.2 25.08,36.2 24.77,35.88 24.77,34.92 26.67,34.92 26.99,35.24 28.89,35.24 29.53,34.61 29.53,33.98 28.89,33.34 26.99,33.34 26.04,34.29 R5.2
D5  (via drill 0.35)
  Top 0.152: v30.48,38.42 31.75,37.15 R6.2
  Bottom 0.152: U2.D5 28.89,38.42 v30.48,38.42
D6  (via drill 0.35)
  Top 0.152: U2.D6 29.84,40.01 29.84,23.5 36.2,17.14 v42.23,17.14 | R1.2 50.8,12.7 50.8,14.29 52.86,16.34 52.86,21.1 53.51,21.75 54.44,21.75 55.56,20.64 U1.2
  Bottom 0.152: v42.23,17.14 42.43,17.14 44.72,14.86 46.1,14.86 R1.2
D7  (via drill 0.35)
  Top 0.152: S4.2 12.7,9.21 12.7,11.11 S1.4 | v25.72,42.23 26.04,41.91 26.04,26.67 26.4,26.3 26.4,17.41 28.57,15.24 28.57,12.7 28.26,12.38 19.68,12.38 19.68,11.43 S1.3
  Bottom 0.152: KEY_80.2 3.49,24.13 2.54,24.13 2.22,23.81 2.22,16.51 7.62,16.51 12.7,11.43 S1.4 13.02,11.43 19.37,11.43 S1.3 | v25.72,42.23 U2.D7
D8  (via drill 0.35)
  Top 0.152: S5.2 25.4,9.21 25.4,11.11 S2.4 | v22.54,46.04 24.13,44.45 24.13,32.8 23.57,32.24 23.57,23.64 24.27,22.94 24.37,22.94 v25.4,21.91
  Bottom 0.152: S2.3 32.07,11.43 25.72,11.43 S2.4 25.4,11.43 v25.4,21.91 | U2.D8 26.67,45.72 22.54,45.72 | 22.54,45.72 6.99,45.72 6.35,45.09 3.17,45.09 2.22,44.13 2.22,42.55 3.81,42.55 4.76,41.59 4.76,40.01 3.17,40.01 2.22,39.05 2.22,37.47 4.76,37.47 KEY_80.3 | 22.54,45.72 v22.54,46.04
D9
  Top 0.152: S6.2 38.1,9.21 38.1,11.11 S3.4
  Bottom 0.152: S3.3 44.77,11.43 38.42,11.43 S3.4 | U2.D9 27.62,49.21 22.11,49.21 21.79,49.53 20.01,49.53 18.9,50.64 18.9,51.26 16.9,53.26 14.75,53.26 14.43,52.95 11.04,52.95 9.27,51.17 5.65,51.17 4.64,50.16 3.17,50.16 1.59,48.58 1.59,36.2 1.91,36.2 | KEY_80.4 1.91,36.2 | S6.2 34.29,5.4 11.75,5.4 1.91,15.24 1.91,36.2
D10  (via drill 0.35)
  Top 0.152: U2.D10 30.48,49.53 v30.48,43.81
  Bottom 0.152: U2.D10 24.13,52.07 JP4.3 | KEY_80.5 6.67,38.1 29.84,38.1 31.11,36.83 33.66,36.83 35.24,38.42 36.51,38.42 37.15,39.05 37.15,43.18 CAN2.3 31.11,43.18 v30.48,43.81
D11
  Top 0.152: U2.D11 31.43,51.12 31.43,39.69 CAN2.5
  Bottom 0.152: U2.D11 28.89,55.56 37.15,55.56 38.1,56.52 48.9,56.52 U3.D11 | KEY_80.6 4.45,39.69 5.4,39.69 5.71,40.01 11.43,40.01 12.06,40.64 30.48,40.64 CAN2.5
D12
  Top 0.152: U2.D12 31.75,53.34 31.75,41.91 CAN2.4
  Bottom 0.152: U2.D12 32.07,57.15 33.34,58.42 37.47,58.42 38.43,57.45 49.02,57.45 49.33,57.15 U3.D12 | KEY_80.7 6.35,40.96 32.7,40.96 CAN2.4
GND  (via drill 0.35)
  Top 0.152: 64.14,10.16 64.14,10.48 X1.3 | 38.42,6.67 S3.2
  Top 0.61: X5.4 X5.6 X5.8 69.49,36.55 68.57,36.55 67.63,37.5 67.63,42.23 C7.2 | S4.1 12.38,5.08 12.7,5.4 | 12.7,5.4 12.94,5.64 S1.2 17.46,11.15 S4.- | 12.7,5.4 16.17,5.4 19.54,2.03 20.46,2.03 23.83,5.4 25.4,5.4 | OK1.5 38.1,41.91 R24.1 IC2.4 38.1,29.52 36.36,27.78 34.45,27.78 33.8,27.13 33.8,26.21 35.56,24.45 U3.GND | C8.2 J1.1 | CAN2.2 37.53,45.72
  Top 0.813: X4.1 X4.M | U1.6 54.61,17.46 U4.1 54.61,10.16 | 54.61,10.16 50.41,10.16 50.16,9.91 48.9,9.91 48.65,10.16 47.62,10.16 47.62,13.97 | C6.2 47.62,13.97 | 47.62,13.97 S6.- 42.86,11.8 42.76,11.7 42.76,11.01 38.42,6.67 | U4.6 54.61,10.16 | SV3.5 SV3.3 64.14,10.16 | S3.2 38.34,5.64 38.1,5.4 | 38.1,5.4 38.1,4.13 S6.1 | 38.1,5.4 36.67,5.4 33.21,1.93 32.2,1.93 28.73,5.4 25.4,5.4 | S5.1 25.08,5.08 25.4,5.4 | 25.4,5.4 25.4,6.39 S2.2 30.06,11.05 30.06,11.7 30.16,11.8 S5.-
  Top 1.016: LED1.K 34.25,58.46 36.76,58.46 37.53,57.69 37.53,45.72 37.53,45.02 OK1.5
  Top 1.27: C8.2 16.92,59.28 16.92,53.75 R7.1 | KEYBRD1.4 69.53,55.71 71.21,54.03 71.21,45.81 C7.2 | C5.2 18.26,21.44 18.26,20.86 17.46,20.06 S4.- | v57.15,22.23 v55.24,24.13
  Bottom 0.152: 76.83,52.07 CAN_GND.2
  Bottom 0.457: SX_GND.2 v55.24,24.13
  Bottom 0.61: X5.8 68.58,34.92 63.02,29.36 63.02,29.26 62.18,28.42 62.08,28.42 57.78,24.13 v55.24,24.13 54.61,24.13 53.34,25.4 53.34,26.67 U3.GND1 48.89,29.21 48.82,29.29 41.83,29.29 40.32,30.8 | X5.4 69.85,29.84 X3.2 | KEYBRD1.4 70.8,55.88 73.34,53.34 77.47,53.34 78.11,52.7 78.11,52.07 | 78.11,52.07 76.83,52.07 | 78.11,52.07 LED_BUS2C.2 | C5.2 17.78,23.5 17.78,24.13 | 17.78,24.13 U2.GND | C9.2 19.05,31.75 | 19.05,31.75 R26.1 25.28,31.75 25.81,31.22 25.93,31.22 U2.GND1 29.37,30.64 36.67,30.64 36.83,30.8 40.32,30.8 | 19.05,31.75 19.05,28.68 17.63,27.26 17.63,26.08 17.78,25.93 17.78,24.13 | IC2.4 40.32,30.8 | KEYBRD.4 8.03,20.32 8.23,20.52 10.91,20.52 S4.- | C7.2 76.2,43.81 SV1.5 | LED1.K 22.3,60.96 22.17,61.09 15.37,61.09 C8.2 | R7.1 13.81,50.64 5.88,50.64 4.13,48.9 KEY_80.14 | v57.15,22.23 57.15,18.1
  Bottom 0.813: X4.M 67.63,14.61 U1.1 57.15,18.1 U1.6 | U4.6 54.77,3.97 59.53,3.97 SV3.5
  pour Bottom: 0,63.5 81.28,63.5 82.55,62.23 82.55,2.54 80.01,0 0,0
LEDS_K_SDA
  Top 0.152: KEYBRD.1 4.76,21.59 4.76,14.92 5.71,13.97 7.62,13.97 7.62,29.84 4.76,32.7 4.76,45.09 KEY_80.11
  Bottom 0.152: R12.2 19.37,46.04 6.35,46.04 KEY_80.11
N$1
  Bottom 0.152: U2.TX0 27.94,18.73 30.32,16.35 30.53,16.35 32.02,14.86 38.48,14.86 39.43,13.91 39.43,12.94 39.99,12.38 41.27,12.38 41.27,15.24 40.96,15.56 40.01,15.56 40.01,17.78 SJ1.2
N$2
  Top 0.152: U1.5 60.33,14.29 64.77,14.29 64.77,13.34 X1.2
  Bottom 0.152: R1.1 51.12,2.22 65.41,2.22 SV3.2 65.41,4.76 65.41,9.21 66.99,9.21 67.31,9.53 67.31,13.02 65.09,13.02 X1.2
N$3
  Bottom 0.152: R26.2 U2.RX1 30.48,21.59 32.58,21.59 34.23,19.95 40.38,19.95 41.49,21.06 44.04,21.06 44.77,20.32 49.53,20.32 U3.TX0
N$4
  Top 0.152: S4.+ 15.24,14.29 15.24,22.86 R4.1
N$5  (via drill 0.35)
  Top 0.152: v25.4,35.56 24.45,36.51 24.45,44.45 24.43,44.46 24.43,45 21.59,47.85 21.59,57.15 JP3.2
  Bottom 0.152: U2.D13 12.7,59.69 JP3.2 | v25.4,35.56 CAN2.6
N$6
  Top 0.152: S5.+ 22.23,19.37 R5.1
N$7
  Bottom 0.152: S6.+ 40.32,14.81 39.7,15.43 39.7,16.18 38.41,17.48 34.58,17.48 33.01,19.05 R6.1
N$8  (via drill 0.35)
  Top 0.152: v41.91,46.04 OK1.6 41.91,26.67 IC2.7 | U3.D2 48.26,29.21 R21.1
  Bottom 0.152: v41.91,46.04 42.86,46.04 43.18,46.35 NO_OPTO.1 | R21.1 43.18,27.94 | 43.18,27.94 SJ_SX2.2 | 43.18,27.94 IC2.7
N$10
  Bottom 0.152: SV1.1 73.98,49.21 73.66,48.9 LED_BUS2A.2
N$11
  Bottom 0.152: U4.2 53.34,12.7 60.01,12.7 | 60.01,12.7 62.55,12.7 62.87,13.02 X1.4 | SV3.4 62.87,4.76 62.87,9.84 60.01,12.7
N$12
  Top 0.61: X2.2 43.5,59.37 B1.AC2 R8.2
N$13
  Bottom 0.61: B1.AC1 47.95,61.92 57.77,61.92 58.1,61.59 X2.M X2.1
N$14  (via drill 0.35)
  Top 0.152: B1.+ 45.72,53.34 45.72,49.85 50.16,45.4 v52.7,45.4
  Top 0.61: C2.1 57.78,45.72 | IC1.IN 57.78,45.72 | 57.78,45.72 C4.1 59.05,38.73 D1.C
  Bottom 0.152: v52.7,45.4 53.02,45.72 IC1.IN
  Bottom 0.61: D1.C 62.12,36.2 63.55,37.62 66.81,37.62 67.91,36.51 71.17,36.51 72.87,34.81 74.14,34.81 74.82,34.13 74.82,33.18 74.14,32.5 73.41,32.5 72.28,31.36 72.28,29.37 71.6,28.69 70.46,28.69 69.81,28.04 68.61,28.04 67.63,29.02 SJ_SX3.2
N$15
  Top 0.152: U2.RST 17.78,26.67 JP4.1
N$16
  Top 0.152: U3.D4 49.53,35.56 49.53,34.92 48.26,33.66 R22.1
  Bottom 0.152: 46.04,32.7 46.35,33.02 R22.1 | 46.04,32.7 43.81,30.48 SJ_SX1.2 | 46.04,32.7 IC2.1
N$17
  Top 0.152: B1.- 58.42,53.34 58.42,48.26
  Top 0.61: C3.2 55.24,30.48 52.63,33.1 52.63,34.21 55.24,36.83 C4.2 55.24,44.5 54.53,45.22 54.53,46.28 IC1.GND 58.42,48.26 59.06,48.26 59.13,48.18 60.25,48.18 60.32,48.26 62.23,48.26 | C2.2 62.23,48.26 | C1.2 62.23,48.26
  Bottom 0.152: C3.2 SX_GND.1 | OK1.3 44.45,53.34 B1.-
N$18  (via drill 0.35)
  Top 0.152: v52.07,19.68 52.07,20.96 52.34,21.22 52.34,21.96 50.8,23.49 U3.RX1
  Bottom 0.152: SJ1.1 40.96,17.78 42.07,18.89 51.28,18.89 v52.07,19.68
N$19
  Bottom 0.152: R3.1 LED1.A
N$20
  Bottom 0.152: U3.D13 34.61,56.2 25.08,56.2 JP3.1
N$21  (via drill 0.35)
  Top 0.152: v44.45,47.31 OK1.2 43.18,52.07 40.64,52.07 R8.1
  Bottom 0.152: v44.45,47.31 43.31,47.31 NO_OPTO.2
N$22
  Top 0.152: LED2.3-GND 9.45,65.68 11.43,65.68 CON1.3
  Bottom 0.152: CON1.3 11.43,65.83 7.62,65.83 C11.2 7.62,65.99 5.18,68.42 | 5.18,68.42 5.18,70.71 C10.2 | 5.18,68.42 2.59,65.83 1.37,65.83 CON2.2
N$23
  Top 0.152: KEYBRD1.8 66.67,47.94 C7.1 66.04,43.18 R14.1
  Bottom 0.152: SJ4.2 64.14,40.96 61.59,40.96 61.28,40.64 60.64,40.64 59.84,41.44 59.84,42.37 60.65,43.18 R14.1
N$24  (via drill 0.35)
  Top 0.152: KEYBRD.2 1.91,26.99 1.91,49.85 v2.86,50.8
  Bottom 0.152: KEYBRD1.1 63.82,55.24 55.24,55.24 54.61,55.88 50.17,55.88 48.9,57.15 38.1,57.15 36.83,55.88 27.31,55.88 25.4,53.97 25.4,53.96 14.58,53.96 14.18,53.56 10.79,53.56 9.3,52.07 5.69,52.07 5.02,51.41 3.56,51.41 2.95,50.8 v2.86,50.8
N$25  (via drill 0.35)
  Top 0.152: KEYBRD.8 7.3,16.51 7.3,28.26 2.22,33.34 2.22,49.21 v3.81,50.8
  Bottom 0.152: KEYBRD1.5 66.67,53.66 49.85,53.66 49.21,54.3 49.21,55.56 48.9,55.88 38.1,55.88 37.15,54.93 37.15,54.29 36.51,53.66 14.71,53.66 14.31,53.26 10.92,53.26 9.21,51.55 5.6,51.55 4.85,50.8 v3.81,50.8
N$26
  Bottom 0.61: X5.2 71.12,26.04 | X5.1 71.12,26.04 | SJ_SX3.1 68.77,26.04 69.22,26.04 | X3.3 69.22,26.04 | 71.12,26.04 69.22,26.04
N$27
  Bottom 0.152: U2.A6 13.97,35.56 15.56,35.56 18.1,33.02 23.06,33.02 23.38,33.34 26.35,33.34 26.67,33.02 29.84,33.02 31.11,34.29 33.34,34.29 34.29,35.24 35.88,35.24 38.42,37.78 51.75,37.78 52.07,37.47 61.59,37.47 64.14,40.01 SJ4.1
N$28
  Bottom 0.152: U3.D10 47.94,49.21 37.78,49.21 36.51,50.48 26.99,50.48 26.04,49.53 22.23,49.53 20.95,50.8 JP4.2
N$29
  Bottom 0.152: LED_BUS2B.2 CAN_GND.1 75.88,52.07 75.88,50.48 77.79,50.48 SV1.2
N$30
  Top 0.152: LED2.2-DOUT 4.57,65.83 7.92,65.83 10.36,68.27 11.43,68.27 CON1.2
N$31
  Top 0.152: LED3.3-GND 23.21,65.68 25.19,65.68 CON4.3
  Bottom 0.152: CON4.3 25.19,65.83 21.38,65.83 C13.2 21.38,65.99 18.95,68.42 | 18.95,68.42 18.95,70.71 C12.2 | 18.95,68.42 16.36,65.83 15.13,65.83 CON3.2
N$32
  Top 0.152: C10.1 2.59,70.86 4.42,69.03 LED2.1-VDD 4.57,69.03 7.16,69.03 8.84,70.71 11.43,70.71 CON1.1
  Bottom 0.152: C11.1 7.62,68.88 9.6,68.88 11.43,70.71 CON1.1
N$33
  Top 0.152: LED2.4-DIN 9.3,68.88 7.47,68.88 6.86,68.27 1.37,68.27 CON2.1
N$34
  Top 0.152: LED3.2-DOUT 18.34,65.83 21.69,65.83 24.13,68.27 25.19,68.27 CON4.2
N$35
  Top 0.152: C12.1 16.36,70.86 18.18,69.03 LED3.1-VDD 18.34,69.03 20.93,69.03 22.6,70.71 25.19,70.71 CON4.1
  Bottom 0.152: C13.1 21.38,68.88 23.36,68.88 25.19,70.71 CON4.1
N$36
  Top 0.152: LED3.4-DIN 23.06,68.88 21.23,68.88 20.62,68.27 15.13,68.27 CON3.1
N$37
  Top 0.152: LED4.4 46.21,65.99 42.7,65.99 42.55,65.83 CON5.2
  Bottom 0.152: CON6.3 52.45,65.83 48.8,65.83 C15.2 48.64,65.99 46.36,68.27 | 46.36,68.27 46.36,70.71 C14.2 | 46.36,68.27 43.92,65.83 42.55,65.83 CON5.2
N$38
  Top 0.152: R23.1 IC2.2 | IC2.6 39.37,26.67 39.37,34.29 R24.2
  Bottom 0.152: R24.2 R23.1
N$39
  Bottom 0.152: SJ_SX1.1 42.55,30.48 40.64,32.38 IC2.3 41.91,34.29 48.58,34.29 49.53,33.34 53.66,33.34 R25.1
N$40
  Top 0.152: LED4.3 46.36,67.81 48.49,67.81 49.25,67.05 51.23,67.05 52.45,68.27 CON6.2
N$41
  Top 0.152: CON6.1 52.61,70.71 49.86,67.97 LED4.2 49.71,67.97 49.56,68.12 47.27,68.12 44.68,70.71 43.77,70.71 C14.1
  Bottom 0.152: CON6.1 50.62,68.88 48.8,68.88 C15.1
N$42
  Top 0.152: IC2.5 R28.1
  Bottom 0.152: IC2.5 38.1,26.04 40.01,27.94 SJ_SX2.1
N$43
  Top 0.152: LED4.1 49.71,66.14 47.58,66.14 46.66,67.05 43.77,67.05 42.55,68.27 CON5.1
N$44
  Top 0.152: LED5.4 59.71,65.99 56.35,65.99 56.2,65.83 CON7.2
  Bottom 0.152: CON8.3 66.11,65.83 62.14,65.83 C17.2 61.99,65.99 60.01,67.97 | 60.01,67.97 60.01,70.71 C16.2 | 60.01,67.97 57.88,65.83 56.2,65.83 CON7.2
N$45
  Top 0.152: LED5.3 59.86,67.81 61.99,67.81 62.75,67.05 64.89,67.05 66.11,68.27 CON8.2
N$46
  Top 0.152: CON8.1 LED5.2 63.21,67.97 63.06,68.12 60.92,68.12 58.33,70.71 57.42,70.71 C16.1
  Bottom 0.152: CON8.1 64.28,68.88 62.14,68.88 C17.1
N$47
  Top 0.152: LED5.1 63.21,66.14 61.08,66.14 60.16,67.05 57.42,67.05 56.2,68.27 CON7.1
N$48
  Top 0.152: LED6.3-GND 37,66 38.5,66 CON10.3 | C18.2 31.5,70.5 34,70.5 34,69.5 34.5,69 32,66.5 29,66.5 29,66 CON9.2
  Bottom 0.152: CON10.3 38.5,66 35.5,66 C19.2 35,66 29,66 CON9.2
N$49
  Top 0.152: NJ1.1 35,71 35,68.5 32.5,66 LED6.2-DOUT
N$50  (via drill 0.35)
  Top 0.152: C18.1 29,70.5 30,69.5 30,69 32,69 LED6.1-VDD 32.5,69 v33.5,69
  Bottom 0.152: CON10.1 38.5,70.5 37,69 35.5,69 C19.1 35,69 v33.5,69
N$51  (via drill 0.35)
  Top 0.152: v36.5,67.5 36.5,69 LED6.4-DIN
  Bottom 0.152: CJ1.1 33.5,71 32,69.5 | 32,69.5 31,68.5 29,68.5 CON9.1 | v36.5,67.5 34,67.5 32,69.5
N$52
  Top 0.152: O4.2 88.31,59.41 89.43,58.3 89.43,52.27 O3.4
  Bottom 0.152: O4.2 90.22,62.28 97.32,62.28 97.32,8.94 92.76,8.94 INP.4
N$54  (via drill 0.35)
  Top 0.152: LED7.4 74.37,65.99 70.1,65.99 69.95,65.84 CON11.2 | v73.3,67.21 73.61,67.51 73.61,70.71 C20.2
  Bottom 0.152: 73.3,65.84 69.95,65.84 CON11.2 | 73.3,65.84 76.81,65.84 C21.2 77,66 80,66 CON12.3 | 73.3,65.84 v73.3,67.21
N$55
  Bottom 0.152: O2.2 85.24,41.32 85.24,32.65 COPY_LED.2
N$56
  Top 0.152: LED7.3 74.52,67.97 74.98,67.97 77.27,70.26 77.27,70.87 NJ2.1
N$57
  Top 0.152: O1.2 89.7,21.52 89.7,18.64 87.15,16.08 87.15,12.6 87.79,11.96 92.86,11.96 93.39,11.42 INP.2
  Bottom 0.152: COPY_LED.3 88.31,32.12 O1.2
N$58
  Top 0.152: O3.2 89.73,49.42 89.73,47.84 90.85,46.73 O2.4
N$59  (via drill 0.35)
  Top 0.152: CON12.1 80.01,70.71 78.03,68.73 78.03,67.97 LED7.2 77.88,67.82 77.27,67.82 v76.81,67.36
  Bottom 0.152: C20.1 71.17,70.71 73.15,68.73 76.81,68.73 C21.1 76.81,68.58 v76.81,67.36
N$60
  Bottom 0.152: COPY_LED.1 86.72,21.64 89.58,21.64 O1.4
N$61  (via drill 0.35)
  Top 0.152: 75.13,66.75 74.98,66.9 73.91,66.9 73.61,66.6 71.48,66.6 69.95,68.12 CON11.1 | 75.13,66.75 75.74,66.14 77.88,66.14 LED7.1 | 75.13,66.75 v78.49,70.1
  Bottom 0.152: v78.49,70.1 77.72,70.87 77.27,70.87 CJ2.1
N$62  (via drill 0.35)
  Top 0.152: v75.59,69.95 76.5,70.87 NJ2.2
  Bottom 0.152: 76.35,70.41 76.35,70.87 CJ2.2 76.35,70.41 | 76.35,70.41 76.96,69.8 77.88,69.8 79.4,68.28 80.01,68.28 CON12.2 | v75.59,69.95 75.89,69.95 76.35,70.41
N$63  (via drill 0.35)
  Top 0.152: NJ1.2 36,71 v37,70 38,70 38,69 38.5,68.5 CON10.2
  Bottom 0.152: v37,70 36.5,70 35.5,71 CJ1.2
PE
  Top 0.152: X3.PE@ X3.PE
POWER2
  Top 0.61: INP.6 90.22,8.94 96.14,8.94 96.14,22.91 | O4.6 96.14,60.37 96.14,50.85 | 96.14,22.91 96.14,41.32 | 96.14,41.32 96.14,50.85 | O3.6 96.14,50.85 | O2.6 96.14,41.32 | O1.6 96.14,22.91
RESET_K  (via drill 0.35)
  Top 0.152: v8.57,19.68 11.11,22.23 11.11,40.32 U2.A3 | v25.08,43.18 24.75,43.51 24.75,45.12 24.13,45.74 24.13,49.53 R3.2
  Bottom 0.152: KEY_80.10 4.76,42.55 12.06,42.55 U2.A3 13.97,43.18 v25.08,43.18 | KEYBRD.6 7.94,19.68 v8.57,19.68 | KEYBRD1.6 68.26,52.07 66.04,52.07 64.77,53.34 48.58,53.34 47.31,52.07 44.13,52.07 43.18,51.12 43.18,49.53 38.1,49.53 36.83,50.8 R3.2
SCL
  Top 0.152: 14.29,36.83 U2.A5 | 14.29,36.83 14.29,42.86 11.75,42.86 11.11,43.5 11.11,49.85 10.16,50.8 6.35,50.8 4.61,49.06 4.61,47.47 KEY_80.12 | 14.29,36.83 R27.1 C9.1
SDA
  Bottom 0.152: R12.1 U2.A4
SX_T0
  Top 0.152: X5.7 72.07,35.24 72.07,35.56 69.53,38.1 X3.1
  Bottom 0.152: R28.2 40.96,23.18 58.74,23.18 69.22,33.66 X5.7
SX_T1
  Top 0.152: X5.5 72.07,29.53 72.07,29.21 71.12,28.26 66.67,28.26 X3.4
  Bottom 0.152: X3.4 65.48,34.37 57.23,34.37 R25.2
V_5V
  Top 0.152: 86.68,48.31 86.68,56.2 O4.1 | 86.68,48.31 86.68,40.42 O2.1 | O3.1 86.68,48.31
  Top 0.61: O2.1 91.44,35.66 91.44,28.94 85.59,23.09 O1.1
  Bottom 1.016: INP.1 88.31,18.46 O1.1
  pour Top: 85.09,71.17 98.11,71.17 98.11,0.05 85.09,0.05
V_GND
  Top 0.152: INP.3 INP.5 | O1.3 O1.5 92.08,21.68 92.08,37.47 O2.5 | O4.3 O4.5 92.08,56.52 92.08,49.62 O3.5 | O2.5 O2.3 | O3.5 O3.3 | O3.5 92.08,46.99 92.08,40.1 O2.5
  Top 1.016: INP.3 O1.3
  pour Bottom: 85.09,69.9 86.36,71.17 97.79,71.17 97.79,0.05 86.36,0.05 85.09,1.32

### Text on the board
Top: Top | +5V
Bottom: Bot | GND | MobaLedLib | 01.08.20
tPlace: + | Normal
bPlace: by Hardi | by Hardi | (100-1.5) | Main Module
tNames: Ver.:1.5 | 3535 | 3535 | 5050 | 5050 | 5050 | 3535 | DCC | LEDs Main / Module | DCC Nano | LEDs 2 | CAN | LEDs Main / Module | LED Nano | Selectrix | LED0 | Ver.:1.5 | GND +5V | by Hardi | MobaLedLib | + | <= | => | L+R / =All | + | Long / =ESC | + | by Hardi | LED / Test | Sim / Inp. | Inp. / Test | LED N | by Hardi
bNames: <- für Alf | 100-1.5-Arduino_fuer_LEDs | 06.08.20

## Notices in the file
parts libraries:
SparkFun-Connectors: Licensing: Creative Commons ShareAlike 4.0 International - https://creativecommons.org/licenses/by-sa/4.0
